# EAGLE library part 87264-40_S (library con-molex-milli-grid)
RECEPTACAL
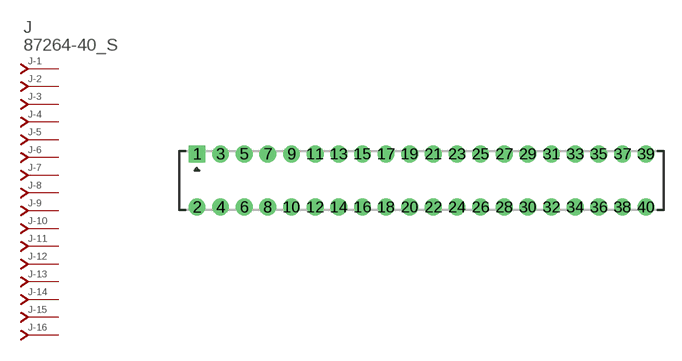
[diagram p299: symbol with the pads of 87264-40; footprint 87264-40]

Designator prefix J; gates -1=J-NV -2=J-N -3=J-N -4=J-N -5=J-N -6=J-N -7=J-N -8=J-N -9=J-N -10=J-N -11=J-N -12=J-N -13=J-N -14=J-N -15=J-N -16=J-N -17=J-N -18=J-N -19=J-N -20=J-N -21=J-N -22=J-N -23=J-N -24=J-N -25=J-N -26=J-N -27=J-N -28=J-N -29=J-N -30=J-N -31=J-N -32=J-N -33=J-N -34=J-N -35=J-N -36=J-N -37=J-N -38=J-N -39=J-N -40=J-N

## 87264-40_S  [87264-40]
1  -1:J  pas
2  -2:J  pas
3  -3:J  pas
4  -4:J  pas
5  -5:J  pas
6  -6:J  pas
7  -7:J  pas
8  -8:J  pas
9  -9:J  pas
10  -10:J  pas
11  -11:J  pas
12  -12:J  pas
13  -13:J  pas
14  -14:J  pas
15  -15:J  pas
16  -16:J  pas
17  -17:J  pas
18  -18:J  pas
19  -19:J  pas
20  -20:J  pas
21  -21:J  pas
22  -22:J  pas
23  -23:J  pas
24  -24:J  pas
25  -25:J  pas
26  -26:J  pas
27  -27:J  pas
28  -28:J  pas
29  -29:J  pas
30  -30:J  pas
31  -31:J  pas
32  -32:J  pas
33  -33:J  pas
34  -34:J  pas
35  -35:J  pas
36  -36:J  pas
37  -37:J  pas
38  -38:J  pas
39  -39:J  pas
40  -40:J  pas

## Footprint 87264-40 (pad centres in mm)
RECEPTACAL Dual Row, Side Entry
drill 0.914 square: 1 -19,2.25
drill 0.914: 2 -19,-2.25; 3 -17,2.25; 4 -17,-2.25; 5 -15,2.25; 6 -15,-2.25; 7 -13,2.25; 8 -13,-2.25; 9 -11,2.25; 10 -11,-2.25; 11 -9,2.25; 12 -9,-2.25; 13 -7,2.25; 14 -7,-2.25; 15 -5,2.25; 16 -5,-2.25; 17 -3,2.25; 18 -3,-2.25; 19 -1,2.25; 20 -1,-2.25; 21 1,2.25; 22 1,-2.25; 23 3,2.25; 24 3,-2.25; 25 5,2.25; 26 5,-2.25; 27 7,2.25; 28 7,-2.25; 29 9,2.25; 30 9,-2.25; 31 11,2.25; 32 11,-2.25; 33 13,2.25; 34 13,-2.25; 35 15,2.25; 36 15,-2.25; 37 17,2.25; 38 17,-2.25; 39 19,2.25; 40 19,-2.25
